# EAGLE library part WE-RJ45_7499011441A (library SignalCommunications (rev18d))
WE-RJ45 LAN Transformer Order Code 7499011441A Design THT xBase-T 10/100 Base-T Ports 1x1 Application Standard Tab Position UP LED (Left-Right) Yellow_Green-Yellow_Green EMI Fingers No Details see: http://katalog.we-online.de/en/pbs/WE-LAN-RJ45 Created by Yingchun Shan 2016 (C) Wurth Elektronik
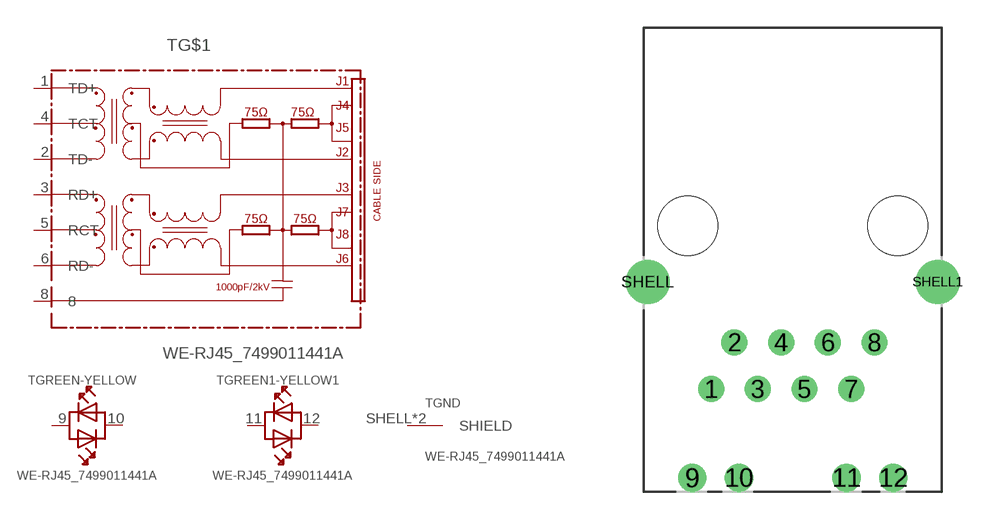
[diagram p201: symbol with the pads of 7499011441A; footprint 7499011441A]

Designator prefix T; gates G$1=7499011441A GREEN-YELLOW=LED_DOUB GREEN1-YELLOW1=LED_DOUB GND=SHIELD

## WE-RJ45_7499011441A  [7499011441A]
1  G$1:TD+
2  G$1:TD-
3  G$1:RD+
4  G$1:TCT
5  G$1:RCT
6  G$1:RD-
8  G$1:8
9  GREEN-YELLOW:AK1  pas
10  GREEN-YELLOW:AK2  pas
11  GREEN1-YELLOW1:AK1  pas
12  GREEN1-YELLOW1:AK2  pas
SHELL  GND:SHIELD  pas
SHELL1  GND:SHIELD  pas

## Footprint 7499011441A (pad centres in mm)
drill 0.9: 1 -4.445,-8.89; 2 -3.175,-6.35; 3 -1.905,-8.89; 4 -0.635,-6.35; 5 0.635,-8.89; 6 1.905,-6.35; 7 3.175,-8.89; 8 4.445,-6.35
drill 1.02: 9 -5.465,-13.72; 10 -2.925,-13.72; 11 2.925,-13.72; 12 5.465,-13.72
drill 1.6: SHELL -7.9,-3.05; SHELL1 7.9,-3.05
hole 3.25 at -5.715,0
hole 3.25 at 5.715,0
